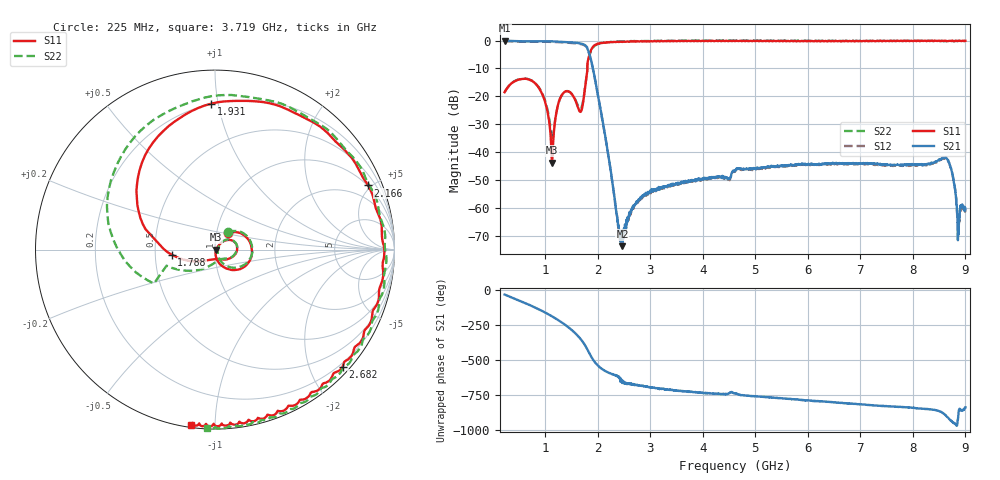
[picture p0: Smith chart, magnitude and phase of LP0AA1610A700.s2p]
!Agilent Technologies,E8358A,US41080443,A.07.50.56
!Agilent E8358A: A.07.50.56
!Date: Wednesday, August 31, 2016 08:54:24
!Correction: S11(Full 2 Port(1,2))
!S21(Full 2 Port(1,2))
!S12(Full 2 Port(1,2))
!S22(Full 2 Port(1,2))
!S2P File: Measurements: S11, S21, S12, S22:
# Hz S  dB  R 50
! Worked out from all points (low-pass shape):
!   1601 points, 225 MHz to 9 GHz, reference 50 ohm
!   highest |S21| = -0.05 dB at 225 MHz (marker M1); lowest = -73.5 dB at 2.468 GHz (marker M2)
!   |S21| within 3 dB of the highest: start of sweep to 1.804 GHz
!   lowest |S11| = -43.6 dB at 1.13 GHz (marker M3), VSWR 1.01, Z = 50.7 - j0.12 ohm
!   |S11| at or under -10 dB: start of sweep to 1.801 GHz
!   |S22| runs from -35.8 to 0.0 dB; largest |S21 - S12| = 0.022
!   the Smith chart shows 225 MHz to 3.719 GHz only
!   S11 on the Smith chart (normalised r, x): 225 MHz: 1.14, +0.22; 1.788 GHz: 0.61, -0.04; 1.931 GHz: 0.20, +0.95; 2.166 GHz: 0.97, +4.79; 2.682 GHz: 0.14, -2.56; 3.719 GHz: 0.01, -0.87
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2.25e8  -18.48 51.5  -0.05 -34.9  -0.24 -34.6  -18.43 53.7
6.911719e8  -13.97 -21.1  -0.30 -107.9  -0.48 -107.6  -13.91 -14.5
9.653906e8  -20.23 -67.3  -0.26 -157.0  -0.45 -156.7  -20.00 -57.4
1.129922e9  -43.63 -10.4  -0.31 169.1  -0.49 169.3  -35.69 -14.5
1.267031e9  -21.38 38.4  -0.42 137.5  -0.60 137.8  -21.49 41.4
1.4535e9  -18.29 -4.0  -0.65 87.5  -0.82 87.8  -18.31 -1.4
1.689328e9  -24.97 -103.4  -1.15 -0.4  -1.33 -0.1  -23.88 -78.0
1.788047e9  -12.29 -173.3  -2.24 -57.6  -2.42 -57.3  -12.34 -153.1
1.930641e9  -1.80 91.5  -12.20 -151.2  -12.38 -150.8  -2.03 118.4
2.166469e9  -0.68 22.7  -36.98 134.1  -37.15 134.3  -0.67 33.7
2.391328e9  -0.51 -12.6  -66.46 95.9  -67.39 94.8  -0.41 -7.2
2.468109e9  -0.50 -21.5  -73.54 62.6  -70.76 56.0  -0.38 -17.2
2.682e9  -0.31 -42.6  -59.55 40.0  -59.63 40.1  -0.20 -39.0
3.153656e9  -0.21 -74.9  -52.94 12.4  -53.28 15.0  -0.09 -70.8
3.718547e9  -0.14 -97.6  -50.56 -10.2  -50.54 -7.1  -0.03 -92.5
4.6125e9  -0.22 -123.2  -46.76 -20.0  -46.85 -21.1  -0.07 -115.5
6.076828e9  -0.14 -163.0  -44.11 -72.2  -44.29 -72.8  -0.05 -152.2
7.541156e9  -0.24 159.5  -44.46 -113.8  -44.70 -113.4  -0.18 162.7
8.627062e9  -0.09 143.8  -41.99 -177.0  -42.15 -176.1  -0.21 135.1
8.747719e9  -0.08 142.7  -47.31 137.7  -47.46 138.6  -0.15 133.6
8.868375e9  -0.11 141.6  -69.45 -172.8  -68.28 -157.9  -0.11 131.8
9e9  -0.12 139.8  -60.25 -119.9  -60.44 -114.7  -0.09 128.9
